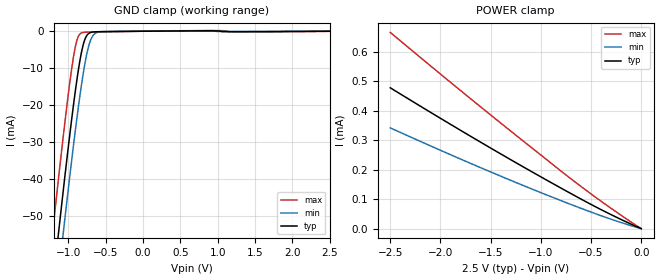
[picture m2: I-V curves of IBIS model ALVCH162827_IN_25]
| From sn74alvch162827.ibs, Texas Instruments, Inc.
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[Model]   ALVCH162827_IN_25
Model_type  Input
Vinl = 0.7
Vinh = 1.7
| variable   typ   min   max
C_comp   5.23pF   4.22pF   6.35pF
[Temperature Range]   40   100   -40
| Ambient temperature   25   85   -40
[Voltage range]   2.5   2.3   2.7
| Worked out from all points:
|   GND clamp passes 1 mA (typ) near -0.75 V on its own axis
[GND Clamp]
| ALVCH162827_IN_25
|   Voltage   I(typ)   I(min)   I(max)
-2.5V     -319.5mA   -330mA     -306.3mA
-1.23V    -72.4mA    -83.89mA   -57.68mA
-1.2V     -66.82mA   -78.32mA   -52.08mA
-1.13V    -53.96mA   -65.46mA   -39.2mA
-1.07V    -43.17mA   -54.63mA   -28.49mA
-925mV    -18.79mA   -29.65mA   -6.062mA
-880mV    -12.23mA   -22.49mA   -2.049mA
-830mV    -6.168mA   -15.15mA   -505.2uA
-780mV    -2.229mA   -8.818mA   -271.3uA
-720mV    -495.6uA   -3.395mA   -227.6uA
-610mV    -137.3uA   -290.5uA   -188.2uA
2.5V      6.664pA    20.75uA    -42.68uA
[POWER Clamp]
| ALVCH162827_IN_25
|   Voltage   I(typ)   I(min)   I(max)
-2.5V     477.5uA    341.6uA    665.3uA
-1.605V   294.2uA    207.5uA    414.3uA
-775mV    133uA      91.85uA    188.8uA
-380mV    61.1uA     41.46uA    88.18uA
-31.15fV  6.664pA    10.41pA    6.889pA
